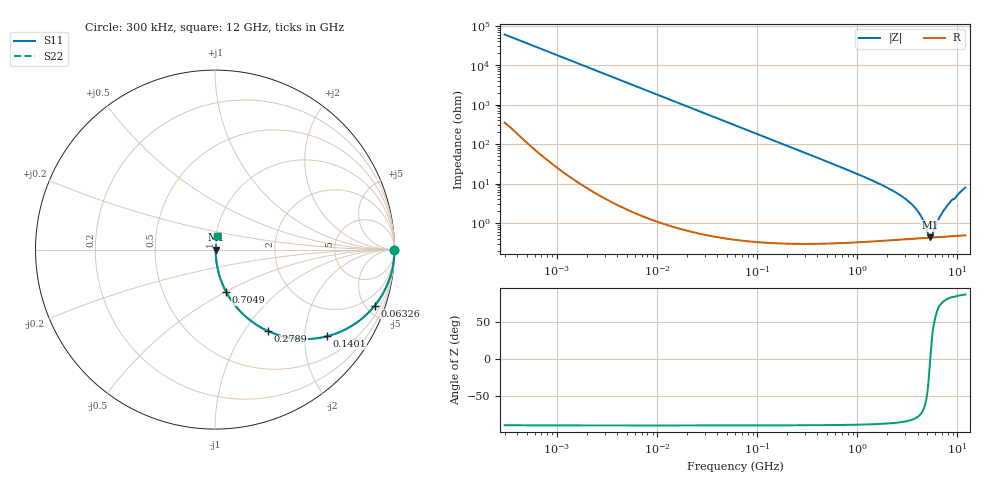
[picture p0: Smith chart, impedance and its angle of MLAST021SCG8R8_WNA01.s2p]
! MLAST021SCG8R8_WNA01  S-PARAMETER MODEL  ( General Type )
! Model Generated by TAIYO YUDEN Corporation (http://www.ty-top.com)
! Version 1.0
! TAIYO YUDEN Control No. 220901
! Copyright(c) 2022 TAIYO YUDEN CO.,LTD. All Rights Reserved.
! Product Description (link to TY-COMPAS)
! https://ds.yuden.co.jp/TYCOMPAS/or/detail?pn=MLAST021SCG8R8CWNA01&u=M
! Products Name : Multilayer Ceramic Capacitors
! Characteristics :
!  Capacitance : 8.8 pF , Rated Voltage : 25V , TCC : CG / C0G
!  Case Size : 0.25 x 0.125 / 0.0098 x 0.0049 [mm/inch] , Thickness : 0.125 / 0.0049 [mm/inch]
!  (Conditions: Temperature = 25 degC , DC Bias Current/Voltage = 0A / 0V)
! External Node Assignments :
!  1  o---| |---o  2
! GND o---------o GND
! Frequency Range : 0.3MHz  -  12000MHz  [ 401 STEP ]
# MHz S RI R 50
! Freq[MHz].  S11 Real  S11 Imag  S21 Real  S21 Imag  S12 Real  S12 Imag  S22 Real  S22 Imag
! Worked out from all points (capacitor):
!   401 points, 300 kHz to 12 GHz, reference 50 ohm
!   read as one part in series: C = 8.8 pF near 316.3 kHz
!   lowest |Z| = 432 mohm at 5.279 GHz (marker M1)
!   series resonance near 5.349 GHz, so ESL is about 100 pH
!   S11 on the Smith chart (normalised r, x): 300 kHz: open; 63.26 MHz: 1.01, -5.72; 140.1 MHz: 1.01, -2.58; 278.9 MHz: 1.01, -1.29; 704.9 MHz: 1.01, -0.50; 12 GHz: 1.01, +0.16
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0.3  1 -0.00166  1.24e-05 0.00166  1.24e-05 0.00166  1 -0.00166
1.769972  0.9999 -0.00979  0.000105 0.00979  0.000105 0.00979  0.9999 -0.00979
10.44266  0.9966 -0.0575  0.00336 0.0575  0.00336 0.0575  0.9966 -0.0575
26.39317  0.979 -0.1429  0.021 0.1429  0.021 0.1429  0.979 -0.1429
60  0.9005 -0.2987  0.0995 0.2987  0.0995 0.2987  0.9005 -0.2987
63.26471  0.8906 -0.3115  0.1094 0.3115  0.1094 0.3115  0.8906 -0.3115
94.13233  0.7863 -0.409  0.2137 0.409  0.2137 0.409  0.7863 -0.409
140.0606  0.6245 -0.4831  0.3755 0.4831  0.3755 0.4831  0.6245 -0.4831
278.9009  0.2957 -0.4541  0.7043 0.4541  0.7043 0.4541  0.2957 -0.4541
353.9943  0.2069 -0.4022  0.7931 0.4022  0.7931 0.4022  0.2069 -0.4022
704.9044  0.0623 -0.2357  0.9377 0.2357  0.9377 0.2357  0.0623 -0.2357
2088.533  0.0089 -0.0724  0.9911 0.0724  0.9911 0.0724  0.0089 -0.0724
2947.191  0.00563 -0.0422  0.9944 0.0422  0.9944 0.0422  0.00563 -0.0422
3740.715  0.00459 -0.0244  0.9954 0.0244  0.9954 0.0244  0.00459 -0.0244
4385.161  0.00429 -0.0133  0.9957 0.0133  0.9957 0.0133  0.00429 -0.0133
5006.236  0.00423 -0.00427  0.9958 0.00427  0.9958 0.00427  0.00423 -0.00427
5278.635  0.00425 -0.000708  0.9958 0.000708  0.9958 0.000708  0.00425 -0.000708
5565.855  0.00429 0.00223  0.9957 -0.00223  0.9957 -0.00223  0.00429 0.00223
6699.894  0.00461 0.014  0.9954 -0.014  0.9954 -0.014  0.00461 0.014
7648.807  0.00507 0.0236  0.9949 -0.0236  0.9949 -0.0236  0.00507 0.0236
8503.825  0.00573 0.0337  0.9943 -0.0337  0.9943 -0.0337  0.00573 0.0337
12000  0.0109 0.0778  0.9891 -0.0778  0.9891 -0.0778  0.0109 0.0778
